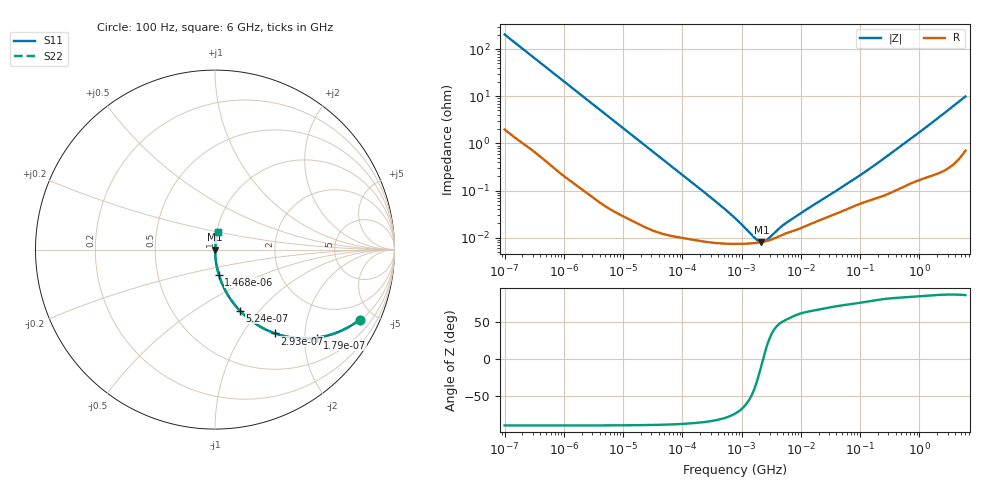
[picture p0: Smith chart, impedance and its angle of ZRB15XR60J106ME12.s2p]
!Murata Part Number: ZRB15XR60J106ME12
!These Parameters are Measured in Series Mode Connection
!Data Generated on Jun 10, 2025
!  o--ll--o
!Port1  Port2
!  o------o
!Operation Temp=25[degC], DC Bias Voltage=0[V]
!Freq. Start=100[Hz] Stop=6[GHz] 401[Steps]
# Hz S RI R 50
!Freq.(Hz) S11(Real) S11(Imag) S21(Real) S21(Imag) S12(Real) S12(Imag) S22(Real) S22(Imag)
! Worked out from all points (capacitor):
!   401 points, 100 Hz to 6 GHz, reference 50 ohm
!   read as one part in series: C = 7.72 uF near 109 Hz
!   lowest |Z| = 8.12 mohm at 2.169 MHz (marker M1)
!   series resonance near 2.307 MHz, so ESL is about 620 pH
!   S11 on the Smith chart (normalised r, x): 100 Hz: 1.04, -4.11; 179 Hz: 1.02, -2.31; 293 Hz: 1.01, -1.41; 524 Hz: 1.01, -0.79; 1.468 kHz: 1.00, -0.28; 6 GHz: 1.01, +0.20
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100  0.8065 -0.3903  0.1935 0.3903  0.1935 0.3903  0.8065 -0.3903
120  0.7456 -0.4308  0.2544 0.4308  0.2544 0.4308  0.7456 -0.4308
179  0.57 -0.4902  0.43 0.4902  0.43 0.4902  0.57 -0.4902
293  0.3347 -0.4669  0.6653 0.4669  0.6653 0.4669  0.3347 -0.4669
524  0.1383 -0.3403  0.8617 0.3403  0.8617 0.3403  0.1383 -0.3403
820  0.0627 -0.2376  0.9373 0.2376  0.9373 0.2376  0.0627 -0.2376
1468  0.0212 -0.1392  0.9788 0.1392  0.9788 0.1392  0.0212 -0.1392
2008  0.0118 -0.103  0.9882 0.103  0.9882 0.103  0.0118 -0.103
6433  0.00145 -0.0327  0.9985 0.0327  0.9985 0.0327  0.00145 -0.0327
40335  0.000155 -0.00529  0.9998 0.00529  0.9998 0.00529  0.000155 -0.00529
316350  7.86e-05 -0.000674  0.9999 0.000674  0.9999 0.000674  7.86e-05 -0.000674
774597  7.36e-05 -0.00025  0.9999 0.00025  0.9999 0.00025  7.36e-05 -0.00025
1585629  7.62e-05 -7.21e-05  0.9999 7.21e-05  0.9999 7.21e-05  7.62e-05 -7.21e-05
2169299  8.04e-05 -1.15e-05  0.9999 1.15e-05  0.9999 1.15e-05  8.04e-05 -1.15e-05
2713602  8.56e-05 3e-05  0.9999 -3e-05  0.9999 -3e-05  8.56e-05 3e-05
3103719  9.01e-05 5.47e-05  0.9999 -5.47e-05  0.9999 -5.47e-05  9.01e-05 5.47e-05
5311619  0.00012 0.000152  0.9999 -0.000152  0.9999 -0.000152  0.00012 0.000152
1.555665e7  0.000201 0.000428  0.9998 -0.000428  0.9998 -0.000428  0.000201 0.000428
9.753859e7  0.00052 0.002  0.9995 -0.002  0.9995 -0.002  0.00052 0.002
3.124326e8  0.0009 0.00575  0.9991 -0.00575  0.9991 -0.00575  0.0009 0.00575
1.873145e9  0.00315 0.0311  0.9968 -0.0311  0.9968 -0.0311  0.00315 0.0311
6e9  0.0165 0.0966  0.9835 -0.0966  0.9835 -0.0966  0.0165 0.0966
